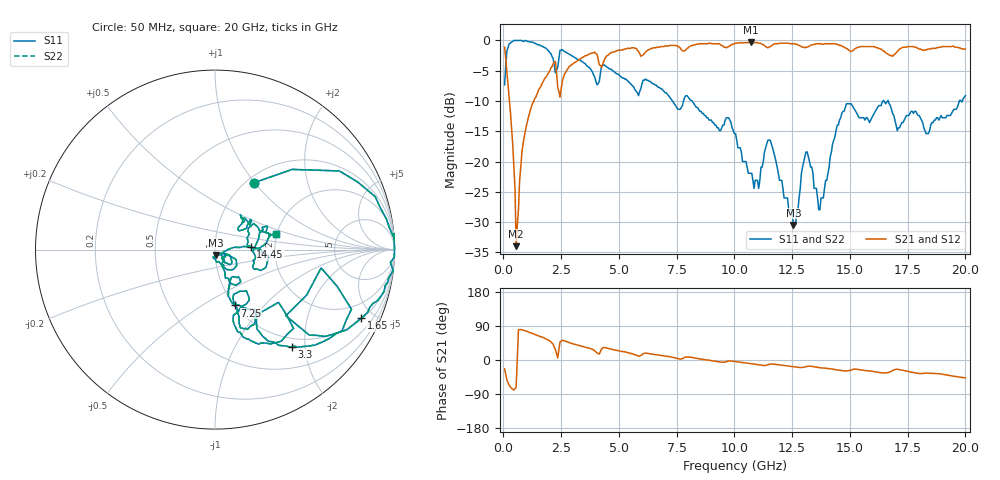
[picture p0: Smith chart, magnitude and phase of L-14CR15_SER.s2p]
#	mhz	s	ma	r	50
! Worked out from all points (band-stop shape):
!   400 points, 50 MHz to 20 GHz, reference 50 ohm
!   highest |S21| = -0.26 dB at 10.7 GHz (marker M1); lowest = -34.0 dB at 550 MHz (marker M2)
!   |S21| within 3 dB of the highest: 3.234 GHz to 4.109 GHz (875.5 MHz wide, 23.8 % of centre); 4.361 GHz to end of sweep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
!   lowest |S11| = -30.5 dB at 12.55 GHz (marker M3), VSWR 1.06, Z = 50.2 - j3 ohm
!   |S11| at or under -10 dB: 7.319 GHz to 7.794 GHz (475.3 MHz wide, 6.29 % of centre); 8.169 GHz to 16.43 GHz (8.263 GHz wide, 67.2 % of centre); 16.66 GHz to 19.74 GHz (3.082 GHz wide, 16.9 % of centre)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
!   |S22| runs from -30.5 to 0.0 dB; largest |S21 - S12| = 0
!   S11 on the Smith chart (normalised r, x): 50 MHz: 1.08, +0.99; 1.65 GHz: 1.05, -4.23; 3.3 GHz: 0.84, -1.74; 7.25 GHz: 1.00, -0.70; 14.45 GHz: 1.50, +0.04; 20 GHz: 1.98, +0.39
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50  0.43 59.9  0.88 -23.2  0.88 -23.2  0.43 59.9
250  0.94 18.3  0.33 -67.2  0.33 -67.2  0.94 18.3
500  1 4.4  0.06 -75.5  0.06 -75.5  1 4.4
550  1 5.1  0.02 -71.7  0.02 -71.7  1 5.1
850  0.98 -4.2  0.14 79.0  0.14 79.0  0.98 -4.2
1650  0.9 -25.2  0.43 60.8  0.43 60.8  0.9 -25.2
2150  0.71 -42.2  0.64 41.6  0.64 41.6  0.71 -42.2
2350  0.6 -9.8  0.41 5.5  0.41 5.5  0.6 -9.8
3300  0.69 -51.8  0.7 38.1  0.7 38.1  0.69 -51.8
3400  0.67 -53.5  0.72 36.6  0.72 36.6  0.67 -53.5
6700  0.41 -71.0  0.88 13.0  0.88 13.0  0.41 -71.0
7250  0.33 -70.6  0.91 8.1  0.91 8.1  0.33 -70.6
10050  0.17 -70.2  0.95 -4.2  0.95 -4.2  0.17 -70.2
10700  0.08 -50.4  0.97 -9.5  0.97 -9.5  0.08 -50.4
11550  0.15 -47.9  0.89 -10.9  0.89 -10.9  0.15 -47.9
12550  0.03 -84.1  0.94 -17.8  0.94 -17.8  0.03 -84.1
13350  0.09 -54.4  0.92 -16.9  0.92 -16.9  0.09 -54.4
13700  0.04 -28.1  0.94 -20.4  0.94 -20.4  0.04 -28.1
14450  0.2 3.6  0.93 -26.3  0.93 -26.3  0.2 3.6
16700  0.3 11.2  0.76 -32.2  0.76 -32.2  0.3 11.2
18400  0.17 41.0  0.85 -34.8  0.85 -34.8  0.17 41.0
20000  0.35 14.2  0.85 -47.1  0.85 -47.1  0.35 14.2
